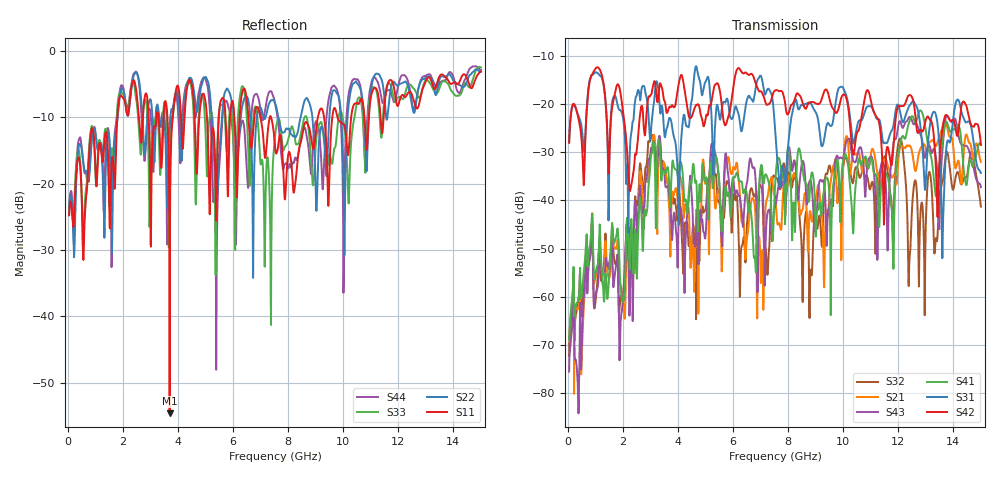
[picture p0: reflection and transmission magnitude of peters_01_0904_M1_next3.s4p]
# MHZ S RI R 50.00
! FREQ  S11  S12  S13  S14
!  S21  S22  S23  S24
!  S31  S32  S33  S34
!  S41  S42  S43  S44
!  REAL  IMAG  REAL  IMAG  REAL  IMAG  REAL  IMAG
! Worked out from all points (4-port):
!   1496 points, 50 MHz to 15 GHz, reference 50 ohm
!   strongest paths, dB at 50 MHz, 3.79 GHz, 7.53 GHz, 11.27 GHz, 15 GHz:
!     S42: -28.0, -20.2, -17.2, -23.2, -28.5
!     S31: -27.9, -24.8, -25.7, -23.1, -34.3
!     S41: -69.0, -32.6, -36.7, -40.2, -28.4
!     S43: -75.6, -48.3, -41.2, -44.4, -37.2
!     S21: -69.3, -38.6, -39.3, -35.4, -32.0
!     S32: -72.2, -39.0, -35.2, -35.6, -41.3
!   lowest |S11| = -54.6 dB at 3.7 GHz (marker M1), VSWR 1.00, Z = 50.2 - j0.0294 ohm
!   |S11| at or under -10 dB: start of sweep to 1.801 GHz; 7.384 GHz to 9.081 GHz (1.697 GHz wide, 20.6 % of centre); 9.792 GHz to 10.29 GHz (497.7 MHz wide, 4.96 % of centre)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
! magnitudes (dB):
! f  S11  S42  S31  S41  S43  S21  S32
! 50 MHz  -24.8  -28.0  -27.9  -69.0  -75.6  -69.3  -72.2
! 2.03 GHz  -7.2  -22.4  -23.7  -60.6  -58.0  -62.1  -60.4
! 3.1 GHz  -12.2  -16.1  -20.7  -27.7  -28.6  -26.9  -26.4
! 3.7 GHz  -54.6  -20.5  -22.9  -38.1  -39.8  -43.9  -40.2
! 5.37 GHz  -21.3  -15.9  -22.7  -31.1  -30.6  -41.7  -34.5
! 6.79 GHz  -9.4  -15.1  -17.7  -51.7  -33.7  -41.0  -39.0
! 15 GHz  -3.1  -28.5  -34.3  -28.4  -37.2  -32.0  -41.3
